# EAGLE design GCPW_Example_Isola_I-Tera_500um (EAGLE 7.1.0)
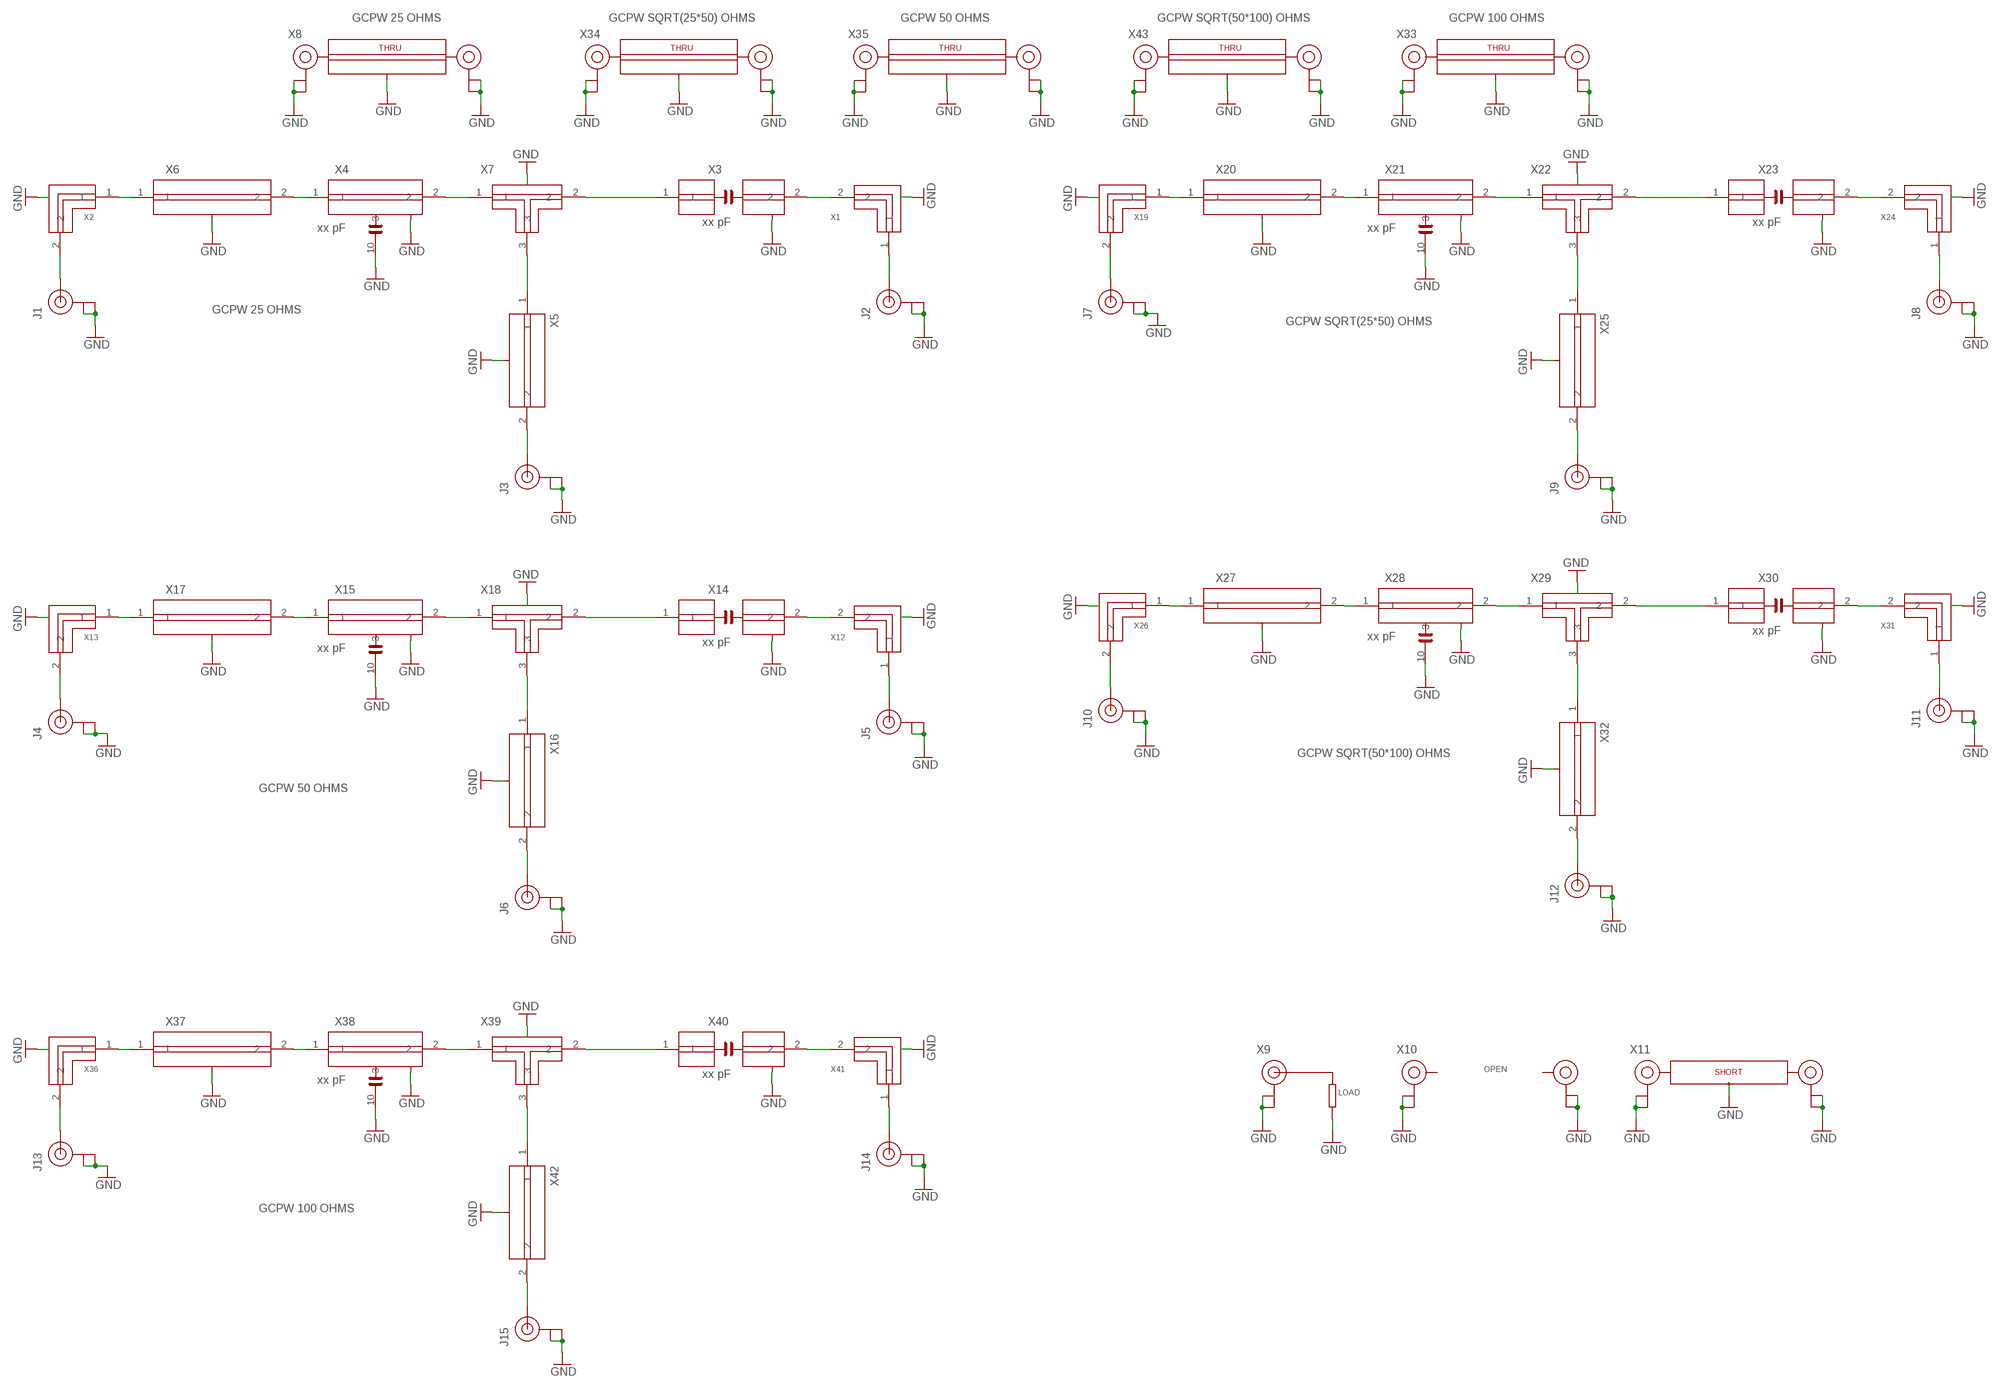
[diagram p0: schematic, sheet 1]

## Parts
J1  U.FL  [U.FL]
J2  U.FL  [U.FL]
J3  U.FL  [U.FL]
J4  U.FL  [U.FL]
J5  U.FL  [U.FL]
J6  U.FL  [U.FL]
J7  U.FL  [U.FL]
J8  U.FL  [U.FL]
J9  U.FL  [U.FL]
J10  U.FL  [U.FL]
J11  U.FL  [U.FL]
J12  U.FL  [U.FL]
J13  U.FL  [U.FL]
J14  U.FL  [U.FL]
J15  U.FL  [U.FL]
X1  CHIPDESIGN_GCPW_25_OHM_L  [GCPW_25_OHM_LEFT]
X2  CHIPDESIGN_GCPW_25_OHM_R  [GCPW_25_OHM_RIGHT]
X3  xx pF  CHIPDESIGN_GCPW_25_OHM_SERIES_0402  [GCPW_25_OHM_0402_SERIES]
X4  xx pF  CHIPDESIGN_GCPW_25_OHM_SHUNT_0402  [GCPW_25_OHM_0402_SHUNT]
X5  CHIPDESIGN_GCPW_25_OHM_TLINE_SHORT  [GCPW_25_OHM_TLINE_SHORT]
X6  CHIPDESIGN_GCPW_25_OHM_TLINE_LONG  [GCPW_25_OHM_TLINE_LONG]
X7  CHIPDESIGN_GCPW_25_OHM_TJUNCTION  [GCPW_25_OHM_TEE]
X8  CHIPDESIGN_GCPW_25_OHM_THRU  [GCPW_25_OHM_THRU]
X9  LOAD_GCPW  [LOAD_GCPW]
X10  OPEN  [OPEN]
X11  SHORT  [SHORT]
X12  CHIPDESIGN_GCPW_50_OHM_L  [GCPW_50_OHM_LEFT]
X13  CHIPDESIGN_GCPW_50_OHM_R  [GCPW_50_OHM_RIGHT]
X14  xx pF  CHIPDESIGN_GCPW_50_OHM_SERIES_0402  [GCPW_50_OHM_0402_SERIES]
X15  xx pF  CHIPDESIGN_GCPW_50_OHM_SHUNT_0402  [GCPW_50_OHM_0402_SHUNT]
X16  CHIPDESIGN_GCPW_50_OHM_TLINE_SHORT  [GCPW_50_OHM_TLINE_SHORT]
X17  CHIPDESIGN_GCPW_50_OHM_TLINE_LONG  [GCPW_50_OHM_TLINE_LONG]
X18  CHIPDESIGN_GCPW_50_OHM_TJUNCTION  [GCPW_50_OHM_TEE]
X19  CHIPDESIGN_GCPW_35_OHM_R  [GCPW_35_OHM_RIGHT]
X20  CHIPDESIGN_GCPW_35_OHM_TLINE_LONG  [GCPW_35_OHM_TLINE_LONG]
X21  xx pF  CHIPDESIGN_GCPW_35_OHM_SHUNT_0402  [GCPW_35_OHM_0402_SHUNT]
X22  CHIPDESIGN_GCPW_35_OHM_TJUNCTION  [GCPW_35_OHM_TEE]
X23  xx pF  CHIPDESIGN_GCPW_35_OHM_SERIES_0402  [GCPW_35_OHM_0402_SERIES]
X24  CHIPDESIGN_GCPW_35_OHM_L  [GCPW_35_OHM_LEFT]
X25  CHIPDESIGN_GCPW_35_OHM_TLINE_SHORT  [GCPW_35_OHM_TLINE_SHORT]
X26  CHIPDESIGN_GCPW_70_OHM_R  [GCPW_70_OHM_RIGHT]
X27  CHIPDESIGN_GCPW_70_OHM_TLINE_LONG  [GCPW_70_OHM_TLINE_LONG]
X28  xx pF  CHIPDESIGN_GCPW_70_OHM_SHUNT_0402  [GCPW_70_OHM_0402_SHUNT]
X29  CHIPDESIGN_GCPW_70_OHM_TJUNCTION  [GCPW_70_OHM_TEE]
X30  xx pF  CHIPDESIGN_GCPW_70_OHM_SERIES_0402  [GCPW_70_OHM_0402_SERIES]
X31  CHIPDESIGN_GCPW_70_OHM_L  [GCPW_70_OHM_LEFT]
X32  CHIPDESIGN_GCPW_70_OHM_TLINE_SHORT  [GCPW_70_OHM_TLINE_SHORT]
X33  CHIPDESIGN_GCPW_100_OHM_THRU  [GCPW_100_OHM_THRU]
X34  CHIPDESIGN_GCPW_35_OHM_THRU  [GCPW_35_OHM_THRU]
X35  CHIPDESIGN_GCPW_50_OHM_THRU  [GCPW_50_OHM_THRU]
X36  CHIPDESIGN_GCPW_100_OHM_R  [GCPW_100_OHM_RIGHT]
X37  CHIPDESIGN_GCPW_100_OHM_TLINE_LONG  [GCPW_100_OHM_TLINE_LONG]
X38  xx pF  CHIPDESIGN_GCPW_100_OHM_SHUNT_0402  [GCPW_100_OHM_0402_SHUNT]
X39  CHIPDESIGN_GCPW_100_OHM_TJUNCTION  [GCPW_100_OHM_TEE]
X40  xx pF  CHIPDESIGN_GCPW_100_OHM_SERIES_0402  [GCPW_100_OHM_0402_SERIES]
X41  CHIPDESIGN_GCPW_100_OHM_L  [GCPW_100_OHM_LEFT]
X42  CHIPDESIGN_GCPW_100_OHM_TLINE_SHORT  [GCPW_100_OHM_TLINE_SHORT]
X43  CHIPDESIGN_GCPW_70_OHM_THRU  [GCPW_70_OHM_THRU]

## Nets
GND: J1.P$1(GND) J1.P$2(GND) J2.P$1(GND) J2.P$2(GND) J3.P$1(GND) J3.P$2(GND) J4.P$1(GND) J4.P$2(GND) J5.P$1(GND) J5.P$2(GND) J6.P$1(GND) J6.P$2(GND) J7.P$1(GND) J7.P$2(GND) J8.P$1(GND) J8.P$2(GND) J9.P$1(GND) J9.P$2(GND) J10.P$1(GND) J10.P$2(GND) J11.P$1(GND) J11.P$2(GND) J12.P$1(GND) J12.P$2(GND) J13.P$1(GND) J13.P$2(GND) J14.P$1(GND) J14.P$2(GND) J15.P$1(GND) J15.P$2(GND) X1.3(GND) X1.4(GND) X1.5(GND) X1.6(GND) X1.7(GND) X2.3(GND) X2.4(GND) X2.5(GND) X2.6(GND) X2.7(GND) X3.3(GND) X3.4(GND) X3.5(GND) X3.6(GND) X3.7(GND) X3.8(GND) X3.9(GND) X3.10(GND) X3.11(GND) X3.12(GND) X4.3(GND) X4.4(GND) X4.5(GND) X4.6(GND) X4.7(GND) X4.8(GND) X4.9(GND) X4.10 X4.11(GND) X4.12(GND) X5.3(GND) X5.4(GND) X5.5(GND) X5.6(GND) X6.3(GND) X6.4(GND) X6.5(GND) X6.6(GND) X6.7(GND) X6.8(GND) X6.9(GND) X6.10(GND) X6.11(GND) X6.12(GND) X7.4(GND) X7.5(GND) X7.6(GND) X7.7(GND) X7.8(GND) X7.9(GND) X7.10(GND) X7.11(GND) X7.12(GND) X8.3(GND) X8.4(GND) X8.5(GND) X8.6(GND) X8.7(GND) X8.8(GND) X8.9(GND) X8.10(GND) X8.11(GND) X8.12(GND) X8.P$1(GND) X8.P$2(GND) X8.P$5(GND) X8.P$6(GND) X9.P$1(GND) X9.P$2(GND) X9.P$6(GND) X9.P$7(GND) X9.P$8(GND) X9.P$9(GND) X9.P$10(GND) X9.P$11(GND) X9.P$12(GND) X10.1(GND) X10.2(GND) X10.3(GND) X10.4(GND) X10.5(GND) X10.6(GND) X10.7(GND) X10.8(GND) X10.9(GND) X10.10(GND) X10.11(GND) X10.12(GND) X10.13(GND) X10.14(GND) X10.15(GND) X10.16(GND) X10.17(GND) X10.18(GND) X10.19(GND) X10.20(GND) X10.21(GND) X10.22(GND) X10.23(GND) X10.24(GND) X11.P$1(GND) X11.P$2(GND) X11.P$3(GND) X11.P$5(GND) X11.P$6(GND) X11.P$7(GND) X12.3(GND) X12.4(GND) X12.5(GND) X12.6(GND) X12.7(GND) X12.8(GND) X12.9(GND) X12.10(GND) X13.3(GND) X13.4(GND) X13.5(GND) X13.6(GND) X13.7(GND) X13.8(GND) X13.9(GND) X13.10(GND) X14.3(GND) X14.4(GND) X14.5(GND) X14.6(GND) X14.7(GND) X14.8(GND) X14.9(GND) X14.10(GND) X14.11(GND) X14.12(GND) X15.3(GND) X15.4(GND) X15.5(GND) X15.6(GND) X15.7(GND) X15.8(GND) X15.9(GND) X15.10 X15.11(GND) X15.12(GND) X16.3(GND) X16.4(GND) X16.5(GND) X16.6(GND) X17.3(GND) X17.4(GND) X17.5(GND) X17.6(GND) X17.7(GND) X17.8(GND) X17.9(GND) X17.10(GND) X17.11(GND) X17.12(GND) X18.4(GND) X18.5(GND) X18.6(GND) X18.7(GND) X18.8(GND) X18.9(GND) X18.10(GND) X18.11(GND) X18.12(GND) X18.13(GND) X18.14(GND) X19.3(GND) X19.4(GND) X19.5(GND) X19.6(GND) X19.7(GND) X20.3(GND) X20.4(GND) X20.5(GND) X20.6(GND) X20.7(GND) X20.8(GND) X20.9(GND) X20.10(GND) X20.11(GND) X20.12(GND) X21.3(GND) X21.4(GND) X21.5(GND) X21.6(GND) X21.7(GND) X21.8(GND) X21.9(GND) X21.10 X21.11(GND) X21.12(GND) X22.4(GND) X22.5(GND) X22.6(GND) X22.7(GND) X22.8(GND) X22.9(GND) X22.10(GND) X22.11(GND) X22.12(GND) X22.13(GND) X22.14(GND) X23.3(GND) X23.4(GND) X23.5(GND) X23.6(GND) X23.7(GND) X23.8(GND) X23.9(GND) X23.10(GND) X23.11(GND) X23.12(GND) X24.3(GND) X24.4(GND) X24.5(GND) X24.6(GND) X24.7(GND) X25.3(GND) X25.4(GND) X25.5(GND) X25.6(GND) X26.3(GND) X26.4(GND) X26.5(GND) X26.6(GND) X26.7(GND) X26.8(GND) X26.9(GND) X26.10(GND) X27.3(GND) X27.4(GND) X27.5(GND) X27.6(GND) X27.7(GND) X27.8(GND) X27.9(GND) X27.10(GND) X27.11(GND) X27.12(GND) X28.3(GND) X28.4(GND) X28.5(GND) X28.6(GND) X28.7(GND) X28.8(GND) X28.9(GND) X28.10 X28.11(GND) X28.12(GND) X29.4(GND) X29.5(GND) X29.6(GND) X29.7(GND) X29.8(GND) X29.9(GND) X29.10(GND) X29.11(GND) X29.12(GND) X29.13(GND) X29.14(GND) X30.3(GND) X30.4(GND) X30.5(GND) X30.6(GND) X30.7(GND) X30.8(GND) X30.9(GND) X30.10(GND) X30.11(GND) X30.12(GND) X31.3(GND) X31.4(GND) X31.5(GND) X31.6(GND) X31.7(GND) X31.8(GND) X31.9(GND) X31.10(GND) X32.3(GND) X32.4(GND) X32.5(GND) X32.6(GND) X33.3(GND) X33.4(GND) X33.5(GND) X33.6(GND) X33.7(GND) X33.8(GND) X33.9(GND) X33.10(GND) X33.11(GND) X33.12(GND) X33.P$1(GND) X33.P$2(GND) X33.P$5(GND) X33.P$6(GND) X34.3(GND) X34.4(GND) X34.5(GND) X34.6(GND) X34.7(GND) X34.8(GND) X34.9(GND) X34.10(GND) X34.11(GND) X34.12(GND) X34.P$1(GND) X34.P$2(GND) X34.P$5(GND) X34.P$6(GND) X35.3(GND) X35.4(GND) X35.5(GND) X35.6(GND) X35.7(GND) X35.8(GND) X35.9(GND) X35.10(GND) X35.11(GND) X35.12(GND) X35.P$1(GND) X35.P$2(GND) X35.P$5(GND) X35.P$6(GND) X36.3(GND) X36.4(GND) X36.5(GND) X36.6(GND) X36.7(GND) X36.8(GND) X36.9(GND) X36.10(GND) X37.3(GND) X37.4(GND) X37.5(GND) X37.6(GND) X37.7(GND) X37.8(GND) X37.9(GND) X37.10(GND) X37.11(GND) X37.12(GND) X38.3(GND) X38.4(GND) X38.5(GND) X38.6(GND) X38.7(GND) X38.8(GND) X38.9(GND) X38.10 X38.11(GND) X38.12(GND) X39.4(GND) X39.5(GND) X39.6(GND) X39.7(GND) X39.8(GND) X39.9(GND) X39.10(GND) X39.11(GND) X39.12(GND) X39.13(GND) X39.14(GND) X40.3(GND) X40.4(GND) X40.5(GND) X40.6(GND) X40.7(GND) X40.8(GND) X40.9(GND) X40.10(GND) X40.11(GND) X40.12(GND) X41.3(GND) X41.4(GND) X41.5(GND) X41.6(GND) X41.7(GND) X41.8(GND) X41.9(GND) X41.10(GND) X42.3(GND) X42.4(GND) X42.5(GND) X42.6(GND) X43.3(GND) X43.4(GND) X43.5(GND) X43.6(GND) X43.7(GND) X43.8(GND) X43.9(GND) X43.10(GND) X43.11(GND) X43.12(GND) X43.P$1(GND) X43.P$2(GND) X43.P$5(GND) X43.P$6(GND)
N$1: J1.P$3(SIGNAL) X2.2
N$2: X2.1 X6.1
N$3: X4.1 X6.2
N$4: X4.2 X7.1
N$5: X3.1 X7.2
N$6: X5.1 X7.3
N$7: J3.P$3(SIGNAL) X5.2
N$8: X1.2 X3.2
N$9: J2.P$3(SIGNAL) X1.1
N$11: J4.P$3(SIGNAL) X13.2
N$12: X13.1 X17.1
N$13: X15.1 X17.2
N$14: X15.2 X18.1
N$15: X14.1 X18.2
N$16: X16.1 X18.3
N$17: J6.P$3(SIGNAL) X16.2
N$18: X12.2 X14.2
N$19: J5.P$3(SIGNAL) X12.1
N$20: J7.P$3(SIGNAL) X19.2
N$21: X19.1 X20.1
N$22: X20.2 X21.1
N$23: X21.2 X22.1
N$24: X22.2 X23.1
N$25: X22.3 X25.1
N$26: J9.P$3(SIGNAL) X25.2
N$27: X23.2 X24.2
N$28: J8.P$3(SIGNAL) X24.1
N$29: J10.P$3(SIGNAL) X26.2
N$30: X26.1 X27.1
N$31: X27.2 X28.1
N$32: X28.2 X29.1
N$33: X29.2 X30.1
N$34: X29.3 X32.1
N$35: J12.P$3(SIGNAL) X32.2
N$36: X30.2 X31.2
N$37: J11.P$3(SIGNAL) X31.1
N$38: J13.P$3(SIGNAL) X36.2
N$39: X36.1 X37.1
N$40: X37.2 X38.1
N$41: X38.2 X39.1
N$42: X39.2 X40.1
N$43: X39.3 X42.1
N$44: J15.P$3(SIGNAL) X42.2
N$45: X40.2 X41.2
N$46: J14.P$3(SIGNAL) X41.1

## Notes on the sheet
- GCPW 25 OHMS | GCPW SQRT(25*50) OHMS | GCPW 50 OHMS | GCPW SQRT(50*100) OHMS | GCPW 100 OHMS
- GCPW 25 OHMS
- GCPW SQRT(25*50) OHMS
- GCPW SQRT(50*100) OHMS
- GCPW 50 OHMS
- GCPW 100 OHMS

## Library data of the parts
J1-J15 = Chipdesign_Isola_050:U.FL: SMD antenna connector- WRL-09144; MPN: U.FL-R-SMT-1(10); OC_NEWARK: 50P8856; PROD_ID: CONN-09193
X1 = Chipdesign_Isola_050:CHIPDESIGN_GCPW_25_OHM_L: Grounded Coplanar Waveguide Line - left; Relative dielectric constant = 3.45; Thickness of dielectric = 0.5mm.; DIELECTRIC: I-TERA-MT-RF; DK: 3.45; E_EFF: 2.753; OC_NEWARK: unknown; PCB_THICKNESS: 0.5MM; ZO: 25 Ohms
X2 = Chipdesign_Isola_050:CHIPDESIGN_GCPW_25_OHM_R: Grounded Coplanar Waveguide Line - right; Relative dielectric constant = 3.45; Thickness of dielectric = 0.5mm.; DIELECTRIC: I-TERA-MT-RF; DK: 3.45; E_EFF: 2.753; OC_NEWARK: unknown; PCB_THICKNESS: 0.5mm; ZO: 25 Ohms
X3 = Chipdesign_Isola_050:CHIPDESIGN_GCPW_25_OHM_SERIES_0402: Grounded Coplanar Waveguide Line - series cap 0402; Relative dielectric constant = 3.45; Thickness of dielectric = 0.5mm.; DIELECTRIC: I-TERA-MT-RF; DK: 3.45; E_EFF: 2.753; OC_NEWARK: unknown; PCB_THICKNESS: 0.5MM; ZO: 25 Ohms
X4 = Chipdesign_Isola_050:CHIPDESIGN_GCPW_25_OHM_SHUNT_0402: Grounded Coplanar Waveguide Line - shunt cap 0402; Relative dielectric constant = 3.45; Thickness of dielectric = 0.5mm.; DIELECTRIC: I-TERA-MT-RF; DK: 3.45; E_EFF: 2.753; OC_NEWARK: unknown; PCB_THICKNESS: 0.5MM; ZO: 25 Ohms
X5 = Chipdesign_Isola_050:CHIPDESIGN_GCPW_25_OHM_TLINE_SHORT: Grounded Coplanar Waveguide Line - TLINE; Relative dielectric constant = 3.45; Thickness of dielectric = 0.5mm.; DIELECTRIC: I-TERA-MT-RF; DK: 3.45; E_EFF: 2.753; OC_NEWARK: unknown; PCB_THICKNESS: 0.5mm; ZO: 25 ohms
X6 = Chipdesign_Isola_050:CHIPDESIGN_GCPW_25_OHM_TLINE_LONG: Grounded Coplanar Waveguide Line - TLINE, long; Relative dielectric constant = 3.45; Thickness of dielectric = 0.5mm.; DIELECTRIC: I-TERA-MT-RF; DK: 3.45; E_EFF: 2.753; OC_NEWARK: unknown; PCB_THICKNESS: 0.5mm; ZO: 25 Ohms
X7 = Chipdesign_Isola_050:CHIPDESIGN_GCPW_25_OHM_TJUNCTION: Grounded Coplanar Waveguide - T JUNCTION, long; Relative dielectric constant = 3.45; Thickness of dielectric = 0.5mm.; DIELECTRIC: I-TERA-MT-RF; DK: 3.45; E_EFF: 2.753; OC_NEWARK: unknown; PCB_THICKNESS: 0.5MM; ZO: 25 Ohms
X8 = Chipdesign_Isola_050:CHIPDESIGN_GCPW_25_OHM_THRU: Relative dielectric constant = 3.45; Thickness of dielectric = 0.5mm.; DIELECTRIC: I-TERA-MT-RF; DK: 3.45; E_EFF: 2.753; OC_NEWARK: unknown; PCB_THICKNESS: 0.5MM; ZO: 25 Ohms
X9 = Chipdesign_Isola_050:LOAD_GCPW: Relative dielectric constant = 3.45; Thickness of dielectric = 0.5mm.; OC_NEWARK: unknown
X10 = Chipdesign_Isola_050:OPEN; OC_NEWARK: unknown
X11 = Chipdesign_Isola_050:SHORT: Relative dielectric constant = 3.45; Thickness of dielectric = 0.5mm.; OC_NEWARK: unknown
X12 = Chipdesign_Isola_050:CHIPDESIGN_GCPW_50_OHM_L: Grounded Coplanar Waveguide Line - left; Relative dielectric constant = 3.45; Thickness of dielectric = 0.5mm.; DIELECTRIC: I-TERA-MT-RF; DK: 3.45; E_EFF: 2.46; OC_NEWARK: unknown; PCB_THICKNESS: 0.5MM; ZO: 50 ohms
X13 = Chipdesign_Isola_050:CHIPDESIGN_GCPW_50_OHM_R: Grounded Coplanar Waveguide Line - right; Relative dielectric constant = 3.45; Thickness of dielectric = 0.5mm.; DIELECTRIC: I-TERA-MT-RF; DK: 3.45; E_EFF: 2.46; OC_NEWARK: unknown; PCB_THICKNESS: 0.5mm; ZO: 50 ohms
X14 = Chipdesign_Isola_050:CHIPDESIGN_GCPW_50_OHM_SERIES_0402: Grounded Coplanar Waveguide Line - series cap 0402; Relative dielectric constant = 3.45; Thickness of dielectric = 0.5mm.; DIELECTRIC: I-TERA-MT-RF; DK: 3.45; E_EFF: 2.46; OC_NEWARK: unknown; PCB_THICKNESS: 0.5MM; ZO: 50 ohms
X15 = Chipdesign_Isola_050:CHIPDESIGN_GCPW_50_OHM_SHUNT_0402: Grounded Coplanar Waveguide Line - shunt cap 0402; Relative dielectric constant = 3.45; Thickness of dielectric = 0.5mm.; DIELECTRIC: I-TERA-MT-RF; DK: 3.45; E_EFF: 2.46; OC_NEWARK: unknown; PCB_THICKNESS: 0.5MM; ZO: 50 ohms
X16 = Chipdesign_Isola_050:CHIPDESIGN_GCPW_50_OHM_TLINE_SHORT: Grounded Coplanar Waveguide Line - TLINE; Relative dielectric constant = 3.45; Thickness of dielectric = 0.5mm.; DIELECTRIC: I-TERA-MT-RF; DK: 3.45; E_EFF: 2.46; OC_NEWARK: unknown; PCB_THICKNESS: 0.5mm; ZO: 50 Ohms
X17 = Chipdesign_Isola_050:CHIPDESIGN_GCPW_50_OHM_TLINE_LONG: Grounded Coplanar Waveguide Line - TLINE, long; Relative dielectric constant = 3.45; Thickness of dielectric = 0.5mm.; DIELECTRIC: I-TERA-MT-RF; DK: 3.45; E_EFF: 2.46; OC_NEWARK: unknown; PCB_THICKNESS: 0.5mm; ZO: 50 ohms
X18 = Chipdesign_Isola_050:CHIPDESIGN_GCPW_50_OHM_TJUNCTION: Grounded Coplanar Waveguide - T JUNCTION, long; Relative dielectric constant = 3.45; Thickness of dielectric = 0.5mm.; DIELECTRIC: I-TERA-MT-RF; DK: 3.45; E_EFF: 2.46; OC_NEWARK: unknown; PCB_THICKNESS: 0.5MM; ZO: 50 ohms
X19 = Chipdesign_Isola_050:CHIPDESIGN_GCPW_35_OHM_R: Grounded Coplanar Waveguide Line - right; Relative dielectric constant = 3.45; Thickness of dielectric = 0.5mm.; DIELECTRIC: I-TERA-MT-RF; DK: 3.45; E_EFF: 2.561; OC_NEWARK: unknown; PCB_THICKNESS: 0.5mm; ZO: sqrt(25*50) Ohms
X20 = Chipdesign_Isola_050:CHIPDESIGN_GCPW_35_OHM_TLINE_LONG: Grounded Coplanar Waveguide Line - TLINE, long; Relative dielectric constant = 3.45; Thickness of dielectric = 0.5mm.; DIELECTRIC: I-TERA-MT-RF; DK: 3.45; E_EFF: 2.561; OC_NEWARK: unknown; PCB_THICKNESS: 0.5mm; ZO: sqrt(25*50) Ohms
X21 = Chipdesign_Isola_050:CHIPDESIGN_GCPW_35_OHM_SHUNT_0402: Grounded Coplanar Waveguide Line - shunt cap 0402; Relative dielectric constant = 3.45; Thickness of dielectric = 0.5mm.; DIELECTRIC: I-TERA-MT-RF; DK: 3.45; E_EFF: 2.561; OC_NEWARK: unknown; PCB_THICKNESS: 0.5MM; ZO: sqrt(25*50) Ohms
X22 = Chipdesign_Isola_050:CHIPDESIGN_GCPW_35_OHM_TJUNCTION: Grounded Coplanar Waveguide - T JUNCTION, long; Relative dielectric constant = 3.45; Thickness of dielectric = 0.5mm.; DIELECTRIC: I-TERA-MT-RF; DK: 3.45; E_EFF: 2.561; OC_NEWARK: unknown; PCB_THICKNESS: 0.5MM; ZO: sqrt(25*50) Ohms
X23 = Chipdesign_Isola_050:CHIPDESIGN_GCPW_35_OHM_SERIES_0402: Grounded Coplanar Waveguide Line - series cap 0402; Relative dielectric constant = 3.45; Thickness of dielectric = 0.5mm.; DIELECTRIC: I-TERA-MT-RF; DK: 3.45; E_EFF: 2.561; OC_NEWARK: unknown; PCB_THICKNESS: 0.5MM; ZO: sqrt(25*50) Ohms
X24 = Chipdesign_Isola_050:CHIPDESIGN_GCPW_35_OHM_L: Grounded Coplanar Waveguide Line - left; Relative dielectric constant = 3.45; Thickness of dielectric = 0.5mm.; DIELECTRIC: I-TERA-MT-RF; DK: 3.45; E_EFF: 2.561; OC_NEWARK: unknown; PCB_THICKNESS: 0.5MM; ZO: sqrt(25*50) Ohms
X25 = Chipdesign_Isola_050:CHIPDESIGN_GCPW_35_OHM_TLINE_SHORT: Grounded Coplanar Waveguide Line - TLINE; Relative dielectric constant = 3.45; Thickness of dielectric = 0.5mm.; DIELECTRIC: I-TERA-MT-RF; DK: 3.45; E_EFF: 2.561; OC_NEWARK: unknown; PCB_THICKNESS: 0.5mm; ZO: sqrt(25*50) Ohms
X26 = Chipdesign_Isola_050:CHIPDESIGN_GCPW_70_OHM_R: Grounded Coplanar Waveguide Line - right; Relative dielectric constant = 3.45; Thickness of dielectric = 0.5mm.; DIELECTRIC: I-TERA-MT-RF; DK: 3.45; E_EFF: 2.34; OC_NEWARK: unknown; PCB_THICKNESS: 0.5MM; ZO: sqrt(50*100) ohms
X27 = Chipdesign_Isola_050:CHIPDESIGN_GCPW_70_OHM_TLINE_LONG: Grounded Coplanar Waveguide Line - TLINE, long; Relative dielectric constant = 3.45; Thickness of dielectric = 0.5mm.; DIELECTRIC: I-TERA-MT-RF; DK: 3.45; E_EFF: 2.34; OC_NEWARK: unknown; PCB_THICKNESS: 0.5MM; ZO: sqrt(50*100) ohms
X28 = Chipdesign_Isola_050:CHIPDESIGN_GCPW_70_OHM_SHUNT_0402: Grounded Coplanar Waveguide Line - shunt cap 0402; Relative dielectric constant = 3.45; Thickness of dielectric = 0.5mm.; DIELECTRIC: I-TERA-MT-RF; DK: 3.45; E_EFF: 2.34; OC_NEWARK: unknown; PCB_THICKNESS: 0.5MM; ZO: sqrt(50*100) ohms
X29 = Chipdesign_Isola_050:CHIPDESIGN_GCPW_70_OHM_TJUNCTION: Grounded Coplanar Waveguide - T JUNCTION, long; Relative dielectric constant = 3.45; Thickness of dielectric = 0.5mm.; DIELECTRIC: I-TERA-MT-RF; DK: 3.45; E_EFF: 2.34; OC_NEWARK: unknown; PCB_THICKNESS: 0.5MM; ZO: sqrt(50*100) ohms
X30 = Chipdesign_Isola_050:CHIPDESIGN_GCPW_70_OHM_SERIES_0402: Grounded Coplanar Waveguide Line - series cap 0402; Relative dielectric constant = 3.45; Thickness of dielectric = 0.5mm.; DIELECTRIC: I-TERA-MT-RF; DK: 3.45; E_EFF: 2.34; OC_NEWARK: unknown; PCB_THICKNESS: 0.5MM; ZO: sqrt(50*100) ohms
X31 = Chipdesign_Isola_050:CHIPDESIGN_GCPW_70_OHM_L: Grounded Coplanar Waveguide Line - left; Relative dielectric constant = 3.45; Thickness of dielectric = 0.5mm.; DIELECTRIC: I-TERA-MT-RF; DK: 3.45; E_EFF: 2.34; OC_NEWARK: unknown; PCB_THICKNESS: 0.5MM; ZO: sqrt(50*100) ohms
X32 = Chipdesign_Isola_050:CHIPDESIGN_GCPW_70_OHM_TLINE_SHORT: Grounded Coplanar Waveguide Line - TLINE; Relative dielectric constant = 3.45; Thickness of dielectric = 0.5mm.; DIELECTRIC: I-TERA-MT-RF; DK: 3.45; E_EFF: 2.34; OC_NEWARK: unknown; PCB_THICKNESS: 0.5mm; ZO: sqrt(50*100) ohms
X33 = Chipdesign_Isola_050:CHIPDESIGN_GCPW_100_OHM_THRU: Relative dielectric constant = 3.45; Thickness of dielectric = 0.5mm.; DIELECTRIC: I-TERA-MT-RF; DK: 3.45; E_EFF: 2.276; OC_NEWARK: unknown; PCB_THICKNESS: 0.5MM; ZO: 100 ohms
X34 = Chipdesign_Isola_050:CHIPDESIGN_GCPW_35_OHM_THRU: Relative dielectric constant = 3.45; Thickness of dielectric = 0.5mm.; DIELECTRIC: I-TERA-MT-RF; DK: 3.45; E_EFF: 2.561; OC_NEWARK: unknown; PCB_THICKNESS: 0.5mm; ZO: sqrt(25*50) Ohms
X35 = Chipdesign_Isola_050:CHIPDESIGN_GCPW_50_OHM_THRU: Relative dielectric constant = 3.45; Thickness of dielectric = 0.5mm.; DIELECTRIC: I-TERA-MT-RF; DK: 3.45; E_EFF: 2.46; OC_NEWARK: unknown; PCB_THICKNESS: 0.5MM; ZO: 50 ohms
X36 = Chipdesign_Isola_050:CHIPDESIGN_GCPW_100_OHM_R: Grounded Coplanar Waveguide Line - right; Relative dielectric constant = 3.45; Thickness of dielectric = 0.5mm.; DIELECTRIC: I-TERA-MT-RF; DK: 3.45; E_EFF: 2.276; OC_NEWARK: unknown; PCB_THICKNESS: 0.5MM; ZO: 100 ohms
X37 = Chipdesign_Isola_050:CHIPDESIGN_GCPW_100_OHM_TLINE_LONG: Grounded Coplanar Waveguide Line - TLINE, long; Relative dielectric constant = 3.45; Thickness of dielectric = 0.5mm.; DIELECTRIC: I-TERA-MT-RF; DK: 3.45; E_EFF: 2.276; OC_NEWARK: unknown; PCB_THICKNESS: 0.5MM; ZO: 100 ohms
X38 = Chipdesign_Isola_050:CHIPDESIGN_GCPW_100_OHM_SHUNT_0402: Grounded Coplanar Waveguide Line - shunt cap 0402; Relative dielectric constant = 3.45; Thickness of dielectric = 0.5mm.; DIELECTRIC: I-TERA-MT-RF; DK: 3.45; E_EFF: 2.276; OC_NEWARK: unknown; PCB_THICKNESS: 0.5MM; ZO: 100 ohms
X39 = Chipdesign_Isola_050:CHIPDESIGN_GCPW_100_OHM_TJUNCTION: Grounded Coplanar Waveguide - T JUNCTION, long; Relative dielectric constant = 3.45; Thickness of dielectric = 0.5mm.; DIELECTRIC: I-TERA-MT-RF; DK: 3.45; E_EFF: 2.276; OC_NEWARK: unknown; PCB_THICKNESS: 0.5MM; ZO: 100 ohms
X40 = Chipdesign_Isola_050:CHIPDESIGN_GCPW_100_OHM_SERIES_0402: Grounded Coplanar Waveguide Line - series cap 0402; Relative dielectric constant = 3.45; Thickness of dielectric = 0.5mm.; DIELECTRIC: I-TERA-MT-RF; DK: 3.45; E_EFF: 2.276; OC_NEWARK: unknown; PCB_THICKNESS: 0.5MM; ZO: 100 ohms
X41 = Chipdesign_Isola_050:CHIPDESIGN_GCPW_100_OHM_L: Grounded Coplanar Waveguide Line - left; Relative dielectric constant = 3.45; Thickness of dielectric = 0.5mm.; DIELECTRIC: I-TERA-MT-RF; DK: 3.45; E_EFF: 2.276; OC_NEWARK: unknown; PCB_THICKNESS: 0.5MM; ZO: 100 ohms
X42 = Chipdesign_Isola_050:CHIPDESIGN_GCPW_100_OHM_TLINE_SHORT: Grounded Coplanar Waveguide Line - TLINE; Relative dielectric constant = 3.45; Thickness of dielectric = 0.5mm.; DIELECTRIC: I-TERA-MT-RF; DK: 3.45; E_EFF: 2.276; OC_NEWARK: unknown; PCB_THICKNESS: 0.5MM; ZO: 100 ohms
X43 = Chipdesign_Isola_050:CHIPDESIGN_GCPW_70_OHM_THRU: Relative dielectric constant = 3.45; Thickness of dielectric = 0.5mm.; DIELECTRIC: I-TERA-MT-RF; DK: 3.45; E_EFF: 2.34; OC_NEWARK: unknown; PCB_THICKNESS: 0.5MM; ZO: sqrt(50*100) ohms

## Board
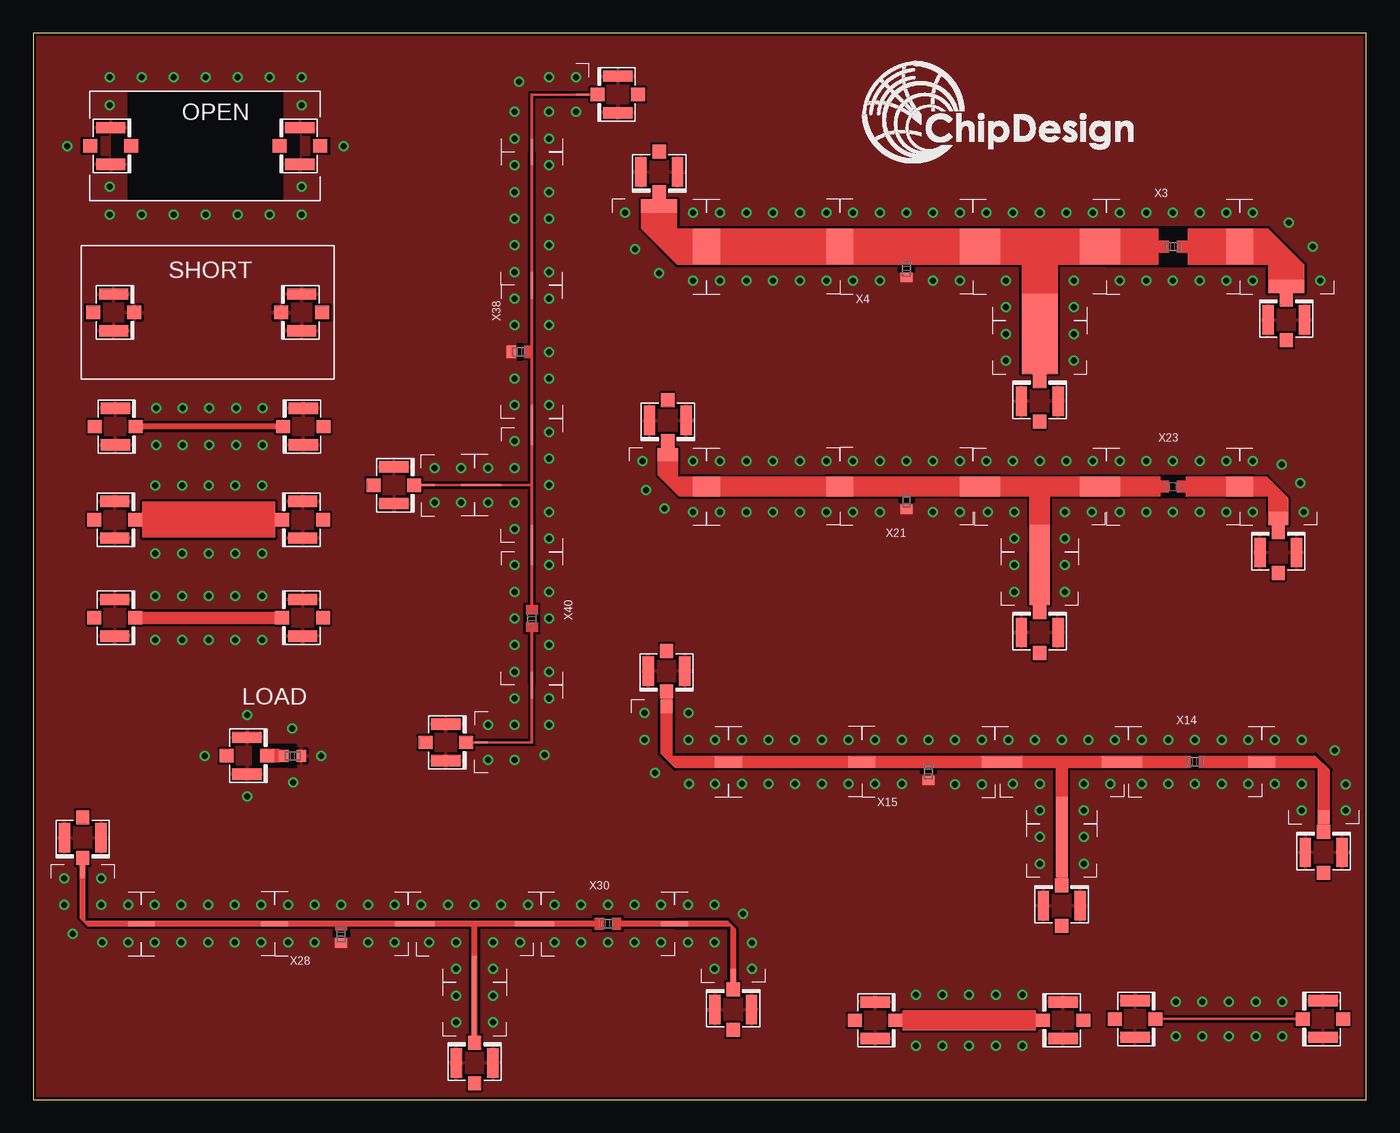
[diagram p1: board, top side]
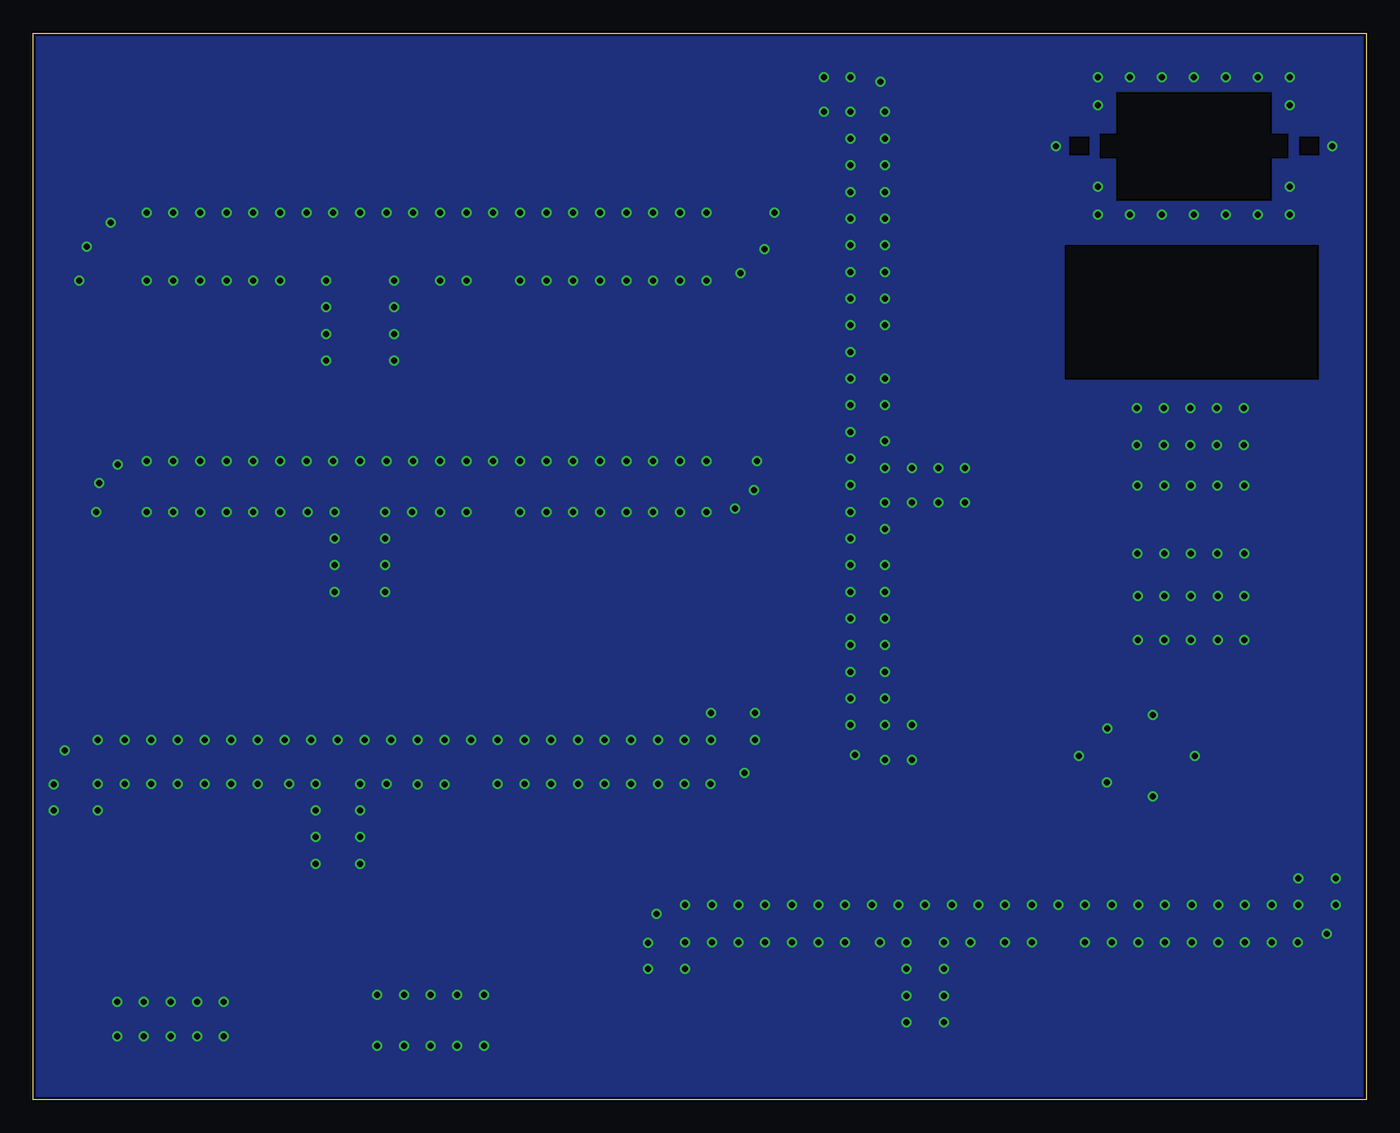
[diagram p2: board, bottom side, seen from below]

Size 100 x 80 mm. Coordinates in mm from the lower left corner, seen from the top.
Outline: 0,0 100,0 100,80 0,80 0,0
Copper layers (1*16): Top 0.035mm / dielectric 1.5mm / Bottom 0.035mm
Design rules "Eagle-DRU - 1506 - LeitOn - 01 and 02 layers - STANDARD": minimum track width 0.15mm, minimum drill 0.3mm, track to track 0.15mm, track to pad 0.15mm, pad to pad 0.15mm, via to via 0.15mm, smd to smd 0.15mm, copper to edge 0.2mm, drill to drill 0.25mm, minimum pad ring 0.15mm, minimum via ring 0.15mm, stop-mask expansion 0.05mm, vias tented up to drill 0mil, thermal gap 0.2mm

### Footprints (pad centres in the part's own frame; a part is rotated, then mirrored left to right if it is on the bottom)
U.FL = smd 2.2 x 0.85: P$1 0,1.375; P$2 0,-1.375 | smd 1.05 x 1: P$3 1.525,0; P$4 -1.525,0
GCPW_25_OHM_LEFT = smd 2.7 x 1: 1 3,-3 | smd 1 x 2.7: 2 0,0 | drill 0.45: 3 0.5,-2.55; 4 0.5,2.55; 5 3.2,1.8; 6 5.55,-2.55; 7 5,0
GCPW_25_OHM_RIGHT = smd 2.7 x 1: 1 -3.05,-3.05 | smd 1 x 2.7: 2 0,0 | drill 0.45: 3 -0.5,-2.55; 4 -0.5,2.55; 5 -3.25,1.8; 6 -5.6,-2.55; 7 -5.05,0
GCPW_25_OHM_0402_SERIES = smd 1 x 2.7: 1 -4.5,0; 2 4.5,0 | drill 0.45: 3 -4,2.55; 4 -2,2.55; 5 -4,-2.55; 6 -2,-2.55; 7 2,2.55; 8 2,-2.55; 9 4,-2.55; 10 4,2.55; 11 0,2.55; 12 0,-2.55
GCPW_25_OHM_0402_SHUNT = smd 1 x 2.7: 1 -4.5,1.65; 2 4.5,1.65 | drill 0.45: 3 -4,4.2; 4 -2,4.2; 5 0,4.2; 6 2,4.2; 7 4,4.2; 8 -4,-0.9; 9 -2,-0.9; 11 2,-0.9; 12 4,-0.9 | smd 0.9 x 0.7: 10 0,-0.65
GCPW_25_OHM_TLINE_SHORT = smd 2 x 2.7: 1 0.5,0; 2 2.5,0 | drill 0.45: 3 0.5,2.55; 4 2.5,2.55; 5 0.5,-2.55; 6 2.5,-2.55
GCPW_25_OHM_TLINE_LONG = smd 1 x 2.7: 1 0,0; 2 9,0 | drill 0.45: 3 0.5,2.55; 4 2.5,2.55; 5 0.5,-2.55; 6 2.5,-2.55; 7 4.5,2.55; 8 4.5,-2.55; 9 6.5,-2.55; 10 6.5,2.55; 11 8.5,2.55; 12 8.5,-2.55
GCPW_25_OHM_TEE = smd 2 x 2.7: 1 -4,4.55; 2 4,4.55 | smd 2.7 x 2: 3 0,0 | drill 0.45: 4 -2.55,2; 5 -2.55,0; 6 2.55,0; 7 2.55,2; 8 4,7.1; 9 2,7.1; 10 0,7.1; 11 -2,7.1; 12 -4,7.1
GCPW_25_OHM_THRU = drill 0.45: 3 0.5,2.55; 4 2.5,2.55; 5 0.5,-2.55; 6 2.5,-2.55; 7 4.5,2.55; 8 4.5,-2.55; 9 6.5,-2.55; 10 6.5,2.55; 11 8.5,2.55; 12 8.5,-2.55 | smd 2.2 x 0.85: P$1 -2.55,1.375; P$2 -2.55,-1.375; P$5 11.55,-1.375; P$6 11.55,1.375 | smd 1.05 x 1: P$3 -1.025,0; P$4 -4.075,0; P$7 10.025,0; P$8 13.075,0
LOAD_GCPW = smd 2.2 x 0.85: P$1 -3.425,1.375; P$2 -3.425,-1.375 | smd 1.05 x 1: P$3 -1.9,0; P$4 -4.95,0 | smd 0.7 x 0.9: P$5 -0.65,0; P$6 0.65,0 | drill 0.45: P$7 2.125,0; P$8 -0.025,2.05; P$9 -3.425,3.05; P$10 -6.6,0; P$11 -3.425,-3.05; P$12 0.025,-2
OPEN = drill 0.45: 1 -1.6,-3.05; 4 -1.6,3.05; 5 12.8,3.05; 8 12.8,-3.05; 9 -1.6,-5.15; 10 0.8,-5.15; 11 3.2,-5.15; 12 5.6,-5.15; 13 8,-5.15; 14 10.4,-5.15; 15 12.8,-5.15; 16 -1.6,5.15; 17 0.8,5.15; 18 3.2,5.15; 19 5.6,5.15; 20 8,5.15; 21 10.4,5.15; 22 12.8,5.15; 23 -4.8,0; 24 15.95,0 | smd 2.2 x 0.85: 2 -1.525,-1.375; 3 -1.525,1.375; 6 12.675,1.375; 7 12.675,-1.375 | smd 1.05 x 1: P$3 0,0; P$4 -3.05,0; P$7 11.15,0; P$8 14.2,0
SHORT = smd 2.2 x 0.85: P$1 -1.55,1.375; P$2 -1.55,-1.375; P$5 12.55,-1.375; P$6 12.55,1.375 | smd 1.05 x 1: P$3 -0.025,0; P$4 -3.075,0; P$7 11.025,0; P$8 14.075,0
GCPW_50_OHM_LEFT = smd 0.9 x 1: 1 4.15,-4.15 | smd 1 x 0.9: 2 0,0 | drill 0.45: 3 2.5,-3.65; 4 2.5,-1.65; 5 0.5,-1.65; 6 0.5,1.65; 7 2.5,1.65; 8 5,0.85; 9 5.8,-1.7; 10 5.8,-3.65
GCPW_50_OHM_RIGHT = smd 0.9 x 1: 1 -4.15,-4.15 | smd 1 x 0.9: 2 0,0 | drill 0.45: 3 -2.5,-3.65; 4 -2.5,-1.65; 5 -0.5,-1.65; 6 -0.5,1.65; 7 -2.5,1.65; 8 -5,0.85; 9 -5.8,-1.7; 10 -5.8,-3.65
GCPW_50_OHM_0402_SERIES = smd 1 x 0.9: 1 -4.5,0; 2 4.5,0 | drill 0.45: 3 -4,1.65; 4 -2,1.65; 5 -4,-1.65; 6 -2,-1.65; 7 2,1.65; 8 2,-1.65; 9 4,-1.65; 10 4,1.65; 11 0,1.65; 12 0,-1.65
GCPW_50_OHM_0402_SHUNT = smd 1 x 0.9: 1 -4.5,0.75; 2 4.5,0.75 | drill 0.45: 3 -4,2.4; 4 -2,2.4; 5 0,2.4; 6 2,2.4; 7 4,2.4; 8 -4,-0.9; 9 -2,-0.9; 11 2,-0.95; 12 4,-0.95 | smd 0.9 x 0.7: 10 0,-0.65
GCPW_50_OHM_TLINE_SHORT = smd 2 x 0.9: 1 0.5,0; 2 2.5,0 | drill 0.45: 3 0.5,1.65; 4 2.5,1.65; 5 0.5,-1.65; 6 2.5,-1.65
GCPW_50_OHM_TLINE_LONG = smd 1 x 0.9: 1 0,0; 2 9,0 | drill 0.45: 3 0.5,1.65; 4 2.5,1.65; 5 0.5,-1.65; 6 2.5,-1.65; 7 4.5,1.65; 8 4.5,-1.65; 9 6.5,-1.65; 10 6.5,1.65; 11 8.5,1.65; 12 8.5,-1.65
GCPW_50_OHM_TEE = smd 2 x 0.9: 1 -4,3.65; 2 4,3.65 | smd 0.9 x 2: 3 0,0 | drill 0.45: 4 -3.65,2; 5 -1.65,2; 6 -1.65,0; 7 1.65,0; 8 1.65,2; 9 3.65,2; 10 4,5.3; 11 2,5.3; 12 0,5.3; 13 -2,5.3; 14 -4,5.3
GCPW_35_OHM_RIGHT = smd 1.525 x 1: 1 -2.4,-2.4 | smd 1 x 1.525: 2 0,0 | drill 0.45: 3 -0.5,-1.9; 4 -0.5,1.9; 5 -4.05,0.25; 6 -4.3,-1.9; 7 -2.65,1.65
GCPW_35_OHM_TLINE_LONG = smd 1 x 1.525: 1 0,0; 2 9,0 | drill 0.45: 3 0.5,1.9; 4 2.5,1.9; 5 0.5,-1.9; 6 2.5,-1.9; 7 4.5,1.9; 8 4.5,-1.9; 9 6.5,-1.9; 10 6.5,1.9; 11 8.5,1.9; 12 8.5,-1.9
GCPW_35_OHM_0402_SHUNT = smd 1 x 1.525: 1 -4.5,1.05; 2 4.5,1.05 | drill 0.45: 3 -4,2.95; 4 -2,2.95; 5 0,2.95; 6 2,2.95; 7 4,2.95; 8 -4,-0.85; 9 -2,-0.85; 11 2,-0.85; 12 4,-0.85 | smd 0.9 x 0.7: 10 0,-0.65
GCPW_35_OHM_TEE = smd 2 x 1.525: 1 -4,3.9; 2 4,3.9 | smd 1.525 x 2: 3 0,0 | drill 0.45: 4 -3.9,2; 5 -1.9,2; 6 -1.9,0; 7 1.9,0; 8 1.9,2; 9 3.9,2; 10 4,5.8; 11 2,5.8; 12 0,5.8; 13 -2,5.8; 14 -4,5.8
GCPW_35_OHM_0402_SERIES = smd 1 x 1.525: 1 -4.5,0; 2 4.5,0 | drill 0.45: 3 -4,1.9; 4 -2,1.9; 5 0,1.9; 6 2,1.9; 7 4,1.9; 8 4,-1.9; 9 2,-1.9; 10 0,-1.9; 11 -2,-1.9; 12 -4,-1.9
GCPW_35_OHM_LEFT = smd 1.525 x 1: 1 2.4,-2.4 | smd 1 x 1.525: 2 0,0 | drill 0.45: 3 0.5,-1.9; 4 0.5,1.9; 5 4.05,0.25; 6 4.3,-1.9; 7 2.65,1.65
GCPW_35_OHM_TLINE_SHORT = smd 2 x 1.525: 1 0.5,0; 2 2.5,0 | drill 0.45: 3 0.5,1.9; 4 2.5,1.9; 5 0.5,-1.9; 6 2.5,-1.9
GCPW_70_OHM_RIGHT = smd 0.415 x 1: 1 -3.9,-3.9 | smd 1 x 0.415: 2 0,0 | drill 0.45: 3 -2.5,-3.4; 4 -2.5,-1.4; 5 -0.5,-1.4; 6 -0.5,1.4; 7 -2.5,1.4; 8 -4.65,0.75; 9 -5.3,-1.45; 10 -5.3,-3.4
GCPW_70_OHM_TLINE_LONG = smd 1 x 0.415: 1 0,0; 2 9,0 | drill 0.45: 3 0.5,1.4; 4 2.5,1.4; 5 0.5,-1.4; 6 2.5,-1.4; 7 4.5,1.4; 8 4.5,-1.4; 9 6.5,-1.4; 10 6.5,1.4; 11 8.5,1.4; 12 8.5,-1.4
GCPW_70_OHM_0402_SHUNT = smd 1 x 0.415: 1 -4.5,0.8; 2 4.5,0.8 | drill 0.45: 3 -4,2.2; 4 -2,2.2; 5 0,2.2; 6 2,2.2; 7 4,2.2; 8 -4,-0.6; 9 -2,-0.6; 11 2,-0.6; 12 4,-0.6 | smd 0.9 x 0.7: 10 0,-0.65
GCPW_70_OHM_TEE = smd 2 x 0.415: 1 -4,3.4; 2 4,3.4 | smd 0.415 x 2: 3 0,0 | drill 0.45: 4 -3.4,2; 5 -1.4,2; 6 -1.4,0; 7 1.4,0; 8 1.4,2; 9 3.4,2; 10 4,4.8; 11 2,4.8; 12 0,4.8; 13 -2,4.8; 14 -4,4.8
GCPW_70_OHM_0402_SERIES = smd 1 x 0.415: 1 -4.5,0; 2 4.5,0 | drill 0.45: 3 -4,1.4; 4 -2,1.4; 5 -4,-1.4; 6 -2,-1.4; 7 2,1.4; 8 2,-1.4; 9 4,-1.4; 10 4,1.4; 11 0,1.4; 12 0,-1.4
GCPW_70_OHM_LEFT = smd 0.415 x 1: 1 3.9,-3.9 | smd 1 x 0.415: 2 0,0 | drill 0.45: 3 2.5,-3.4; 4 2.5,-1.4; 5 0.5,-1.4; 6 0.5,1.4; 7 2.5,1.4; 8 4.65,0.75; 9 5.3,-1.45; 10 5.3,-3.4
GCPW_70_OHM_TLINE_SHORT = smd 2 x 0.415: 1 0.5,0; 2 2.5,0 | drill 0.45: 3 0.5,1.4; 4 2.5,1.4; 5 0.5,-1.4; 6 2.5,-1.4
GCPW_100_OHM_THRU = drill 0.45: 3 0.5,1.3; 4 2.5,1.3; 5 0.5,-1.3; 6 2.5,-1.3; 7 4.5,1.3; 8 4.5,-1.3; 9 6.5,-1.3; 10 6.5,1.3; 11 8.5,1.3; 12 8.5,-1.3 | smd 2.2 x 0.85: P$1 -2.55,1.375; P$2 -2.55,-1.375; P$5 11.55,-1.375; P$6 11.55,1.375 | smd 1.05 x 1: P$3 -1.025,0; P$4 -4.075,0; P$7 10.025,0; P$8 13.075,0
GCPW_35_OHM_THRU = drill 0.45: 3 0.5,1.9; 4 2.5,1.9; 5 0.5,-1.9; 6 2.5,-1.9; 7 4.5,1.9; 8 4.5,-1.9; 9 6.5,-1.9; 10 6.5,1.9; 11 8.5,1.9; 12 8.5,-1.9 | smd 2.2 x 0.85: P$1 -2.55,1.375; P$2 -2.55,-1.375; P$5 11.55,-1.375; P$6 11.55,1.375 | smd 1.05 x 1: P$3 -1.025,0; P$4 -4.075,0; P$7 10.025,0; P$8 13.075,0
GCPW_50_OHM_THRU = drill 0.45: 3 0.5,1.65; 4 2.5,1.65; 5 0.5,-1.65; 6 2.5,-1.65; 7 4.5,1.65; 8 4.5,-1.65; 9 6.5,-1.65; 10 6.5,1.65; 11 8.5,1.65; 12 8.5,-1.65 | smd 2.2 x 0.85: P$1 -2.55,1.375; P$2 -2.55,-1.375; P$5 11.55,-1.375; P$6 11.55,1.375 | smd 1.05 x 1: P$3 -1.025,0; P$4 -4.075,0; P$7 10.025,0; P$8 13.075,0
GCPW_100_OHM_RIGHT = smd 0.16 x 1: 1 -3.8,-3.8 | smd 1 x 0.16: 2 0,0 | drill 0.45: 3 -2.5,-3.3; 4 -2.5,-1.3; 5 -0.5,-1.3; 6 -0.5,1.3; 7 -2.5,1.3; 8 -4.75,0.95; 9 -5.1,-1.3; 10 -5.1,-3.3
GCPW_100_OHM_TLINE_LONG = smd 1 x 0.16: 1 0,0; 2 9,0 | drill 0.45: 3 0.5,1.3; 4 2.5,1.3; 5 0.5,-1.3; 6 2.5,-1.3; 7 4.5,1.3; 8 4.5,-1.3; 9 6.5,-1.3; 10 6.5,1.3; 11 8.5,1.3; 12 8.5,-1.3
GCPW_100_OHM_0402_SHUNT = smd 1 x 0.16: 1 -4.5,0.9; 2 4.5,0.9 | drill 0.45: 3 -4,2.2; 4 -2,2.2; 5 0,2.2; 6 2,2.2; 7 4,2.2; 8 -4,-0.4; 9 -2,-0.4; 11 2,-0.4; 12 4,-0.4 | smd 0.9 x 0.7: 10 0,-0.65
GCPW_100_OHM_TEE = smd 2 x 0.16: 1 -4,3.3; 2 4,3.3 | smd 0.16 x 2: 3 0,0 | drill 0.45: 4 -3.3,2; 5 -1.3,2; 6 -1.3,0; 7 1.3,0; 8 1.3,2; 9 3.3,2; 10 4,4.6; 11 2,4.6; 12 0,4.6; 13 -2,4.6; 14 -4,4.6
GCPW_100_OHM_0402_SERIES = smd 1 x 0.16: 1 -4.5,0; 2 4.5,0 | drill 0.45: 3 -4,1.3; 4 -2,1.3; 5 -4,-1.3; 6 -2,-1.3; 7 2,1.3; 8 2,-1.3; 9 4,-1.3; 10 4,1.3; 11 0,1.3; 12 0,-1.3
GCPW_100_OHM_LEFT = smd 0.16 x 1: 1 3.8,-3.8 | smd 1 x 0.16: 2 0,0 | drill 0.45: 3 2.5,-3.3; 4 2.5,-1.3; 5 0.5,-1.3; 6 0.5,1.3; 7 2.5,1.3; 8 4.75,0.95; 9 5.1,-1.3; 10 5.1,-3.3
GCPW_100_OHM_TLINE_SHORT = smd 1 x 0.16: 1 0,0; 2 3,0 | drill 0.45: 3 0.5,1.3; 4 2.5,1.3; 5 0.5,-1.3; 6 2.5,-1.3
GCPW_70_OHM_THRU = drill 0.45: 3 0.5,1.4; 4 2.5,1.4; 5 0.5,-1.4; 6 2.5,-1.4; 7 4.5,1.4; 8 4.5,-1.4; 9 6.5,-1.4; 10 6.5,1.4; 11 8.5,1.4; 12 8.5,-1.4 | smd 2.2 x 0.85: P$1 -2.55,1.375; P$2 -2.55,-1.375; P$5 11.55,-1.375; P$6 11.55,1.375 | smd 1.05 x 1: P$3 -1.025,0; P$4 -4.075,0; P$7 10.025,0; P$8 13.075,0

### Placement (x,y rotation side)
J1  46.95,69.6 270 top
J2  94,58.5 90 top
J3  75.5,52.4 90 top
J4  47.5,32.15 270 top
J5  96.8,18.55 90 top
J6  77.15,14.55 90 top
J7  47.6,50.95 270 top
J8  93.4,41.05 90 top
J9  75.5,35.05 90 top
J10  3.7,19.65 270 top
J11  52.5,6.75 90 top
J12  33.1,2.75 90 top
J13  43.85,75.4 180 top
J14  30.95,26.8 0 top
J15  27.05,46.1 0 top
X1  91,64 0 top
X2  46.95,67.05 90 top
X3  85.5,64 0 top
X4  65.5,62.35 0 top
X5  75.5,57.95 270 top
X6  51,64 0 top
X7  75.5,59.45 0 top
X8  8.66,43.51 0 top
X9  19.45,25.79 0 top
X10  7.33,71.55 0 top
X11  7.58,59.06 0 top
X12  92.65,25.35 0 top
X13  47.5,29.5 90 top
X14  87.15,25.35 0 top
X15  67.15,24.6 0 top
X16  77.15,20.2 270 top
X17  52.65,25.35 0 top
X18  77.15,21.7 0 top
X19  47.6,48.4 90 top
X20  51,46 0 top
X21  65.5,44.95 0 top
X22  75.5,42.1 0 top
X23  85.5,46 0 top
X24  91,46 0 top
X25  75.5,40.6 270 top
X26  3.7,17.1 90 top
X27  8.6,13.2 0 top
X28  23.1,12.4 0 top
X29  33.1,9.8 0 top
X30  43.1,13.2 0 top
X31  48.6,13.2 0 top
X32  33.1,8.3 270 top
X33  94.2,6.05 180 top
X34  65.7,5.95 0 top
X35  8.65,36.15 0 top
X36  41.2,75.4 0 top
X37  37.4,70.6 270 top
X38  36.5,56.1 270 top
X39  34.1,46.1 270 top
X40  37.4,36.1 270 top
X41  37.4,30.6 270 top
X42  32.6,46.1 180 top
X43  8.7,50.5 0 top

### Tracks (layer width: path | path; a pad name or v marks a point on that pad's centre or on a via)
GND
  pour Top: 0,0 100,0 100,80 0,80
  pour Bottom: 0,0 100,0 100,80 0,80
N$1
  Top 0.15: J1.P$3 46.96,67.92 46.96,67.11 X2.2
N$2
  Top 0.15: X2.1 50.05,64.03 50.86,64.03 X6.1
N$3
  Top 0.15: X6.2 60.12,64.03 60.94,64.03 X4.1
N$4
  Top 0.15: X4.2 70.04,64.03 71.5,64.03 X7.1
N$5
  Top 0.15: X7.2 79.62,64.03 80.92,64.03 X3.1
N$6
  Top 0.15: X5.1 75.56,57.52 75.56,59.31 X7.3
N$7
  Top 0.15: J3.P$3 75.56,53.95 75.56,55.41 X5.2
N$8
  Top 0.15: X3.2 90.03,64.03 90.84,64.03 X1.2
N$9
  Top 0.15: J2.P$3 94.09,60.12 94.09,60.94 X1.1
N$11
  Top 0.15: 47.5,29.57 X13.2 | 47.5,30.39 J4.P$3
  Top 0.9: 47.5,30.39 47.5,29.57
N$12
  Top 0.15: X17.1 X13.1
N$13
  Top 0.15: X15.1 X17.2
N$14
  Top 0.15: X18.1 X15.2
N$15
  Top 0.15: X18.2 X14.1
N$16
  Top 0.15: X16.1 77.19,19.82 77.19,21.61 X18.3
N$17
  Top 0.15: 77.15,16.25 J6.P$3 | 77.15,17.55 X16.2
  Top 0.9: 77.15,17.55 77.15,16.25
N$18
  Top 0.15: X12.2 X14.2
N$19
  Top 0.15: 96.8,21.12 X12.1 | 96.8,20.31 J5.P$3
  Top 0.9: 96.8,20.31 96.8,21.12
N$20
  Top 0.15: J7.P$3 47.61,49.4 47.61,48.42 X19.2
N$21
  Top 0.15: X19.1 50.05,45.99 50.86,45.99 X20.1
N$22
  Top 0.15: X20.2 60.12,45.99 60.94,45.99 X21.1
N$23
  Top 0.15: X21.2 70.04,45.99 71.5,45.99 X22.1
N$24
  Top 0.15: X23.1 80.92,45.99 79.62,45.99 X22.2
N$25
  Top 0.15: X25.1 75.56,40.14 75.56,42.09 X22.3
N$26
  Top 0.15: J9.P$3 75.56,36.73 75.56,38.02 X25.2
N$27
  Top 0.15: X23.2 90.03,45.99 91,45.99 X24.2
N$28
  Top 0.15: J8.P$3 93.44,42.58 93.44,43.55 X24.1
N$29
  Top 0.15: X26.2 3.74,17.23 3.74,18.04 J10.P$3
N$30
  Top 0.15: X26.1 7.64,13.32 8.45,13.32 X27.1
N$31
  Top 0.15: X27.2 17.71,13.32 18.52,13.32 X28.1
N$32
  Top 0.15: X28.2 27.62,13.32 29.09,13.32 X29.1
N$33
  Top 0.15: X30.1 38.51,13.32 37.21,13.32 X29.2
N$34
  Top 0.15: X32.1 33.15,7.8 33.15,9.75 X29.3
N$35
  Top 0.15: J12.P$3 33.15,4.39 33.15,5.69 X32.2
N$36
  Top 0.15: X30.2 47.61,13.32 48.59,13.32 X31.2
N$37
  Top 0.15: X31.1 52.49,9.26 52.49,8.29 J11.P$3
N$38
  Top 0.16: J13.P$3 X36.2
N$39
  Top 0.1: X36.1 X37.1
N$40
  Top 0.1: X37.2 X38.1
N$41
  Top 0.1: X38.2 X39.1
N$42
  Top 0.1: X39.2 X40.1
N$43
  Top 0.1: X42.1 X39.3
N$44
  Top 0.1: J15.P$3 X42.2
N$45
  Top 0.1: X40.2 X41.2
N$46
  Top 0.16: J14.P$3 X41.1

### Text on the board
tDocu: GCPW 100 OHM | GCPW 25 OHM | GCPW SQRT(25*50) OHM | GCPW 50 OHM | GCPW SQRT(50*100) OHM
